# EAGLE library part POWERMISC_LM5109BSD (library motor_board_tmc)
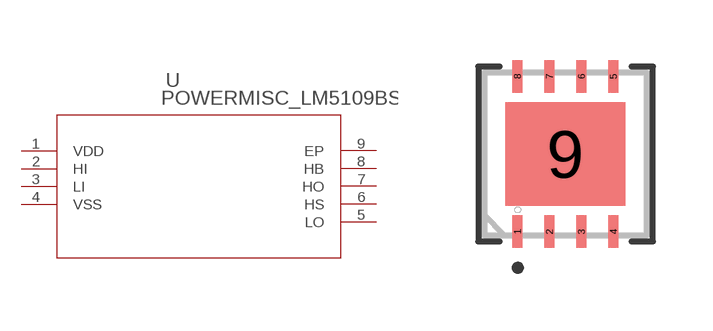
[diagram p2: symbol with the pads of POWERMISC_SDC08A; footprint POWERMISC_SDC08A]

Designator prefix U

## POWERMISC_LM5109BSD (MANUFACTURER_PART_NUMBER: lm5109bsd; VENDOR: Texas Instruments)  [POWERMISC_SDC08A]
1  VDD  pwr
2  HI  in
3  LI  in
4  VSS  pwr
5  LO  out
6  HS  in
7  HO  out
8  HB  in
9  EP  pwr

## Footprint POWERMISC_SDC08A (pad centres in mm)
smd 0.254 x 0.813: 1 -1.2,-1.943; 2 -0.4,-1.943; 3 0.4,-1.943; 4 1.2,-1.943; 5 1.2,1.943; 6 0.4,1.943; 7 -0.4,1.943; 8 -1.2,1.943
smd 2.997 x 2.591: 9 0,0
